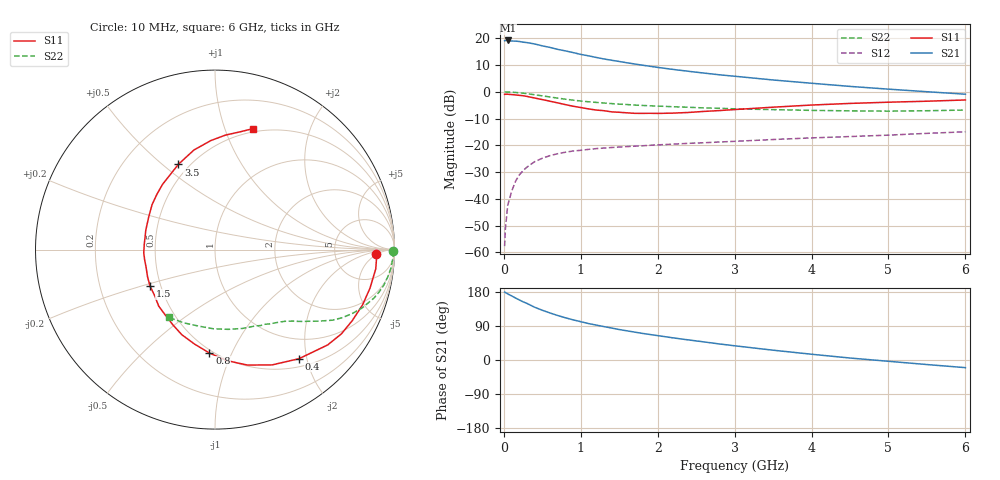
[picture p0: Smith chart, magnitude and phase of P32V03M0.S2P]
! SIEMENS Small Signal Semiconductors
! BFP181
! Si NPN RF Bipolar Junction Transistor in SOT143
! VCE = 2 V  IC = 3 mA
! Common Emitter S-Parameters:  March  1996
# GHz  S  MA  R  50
!  f  S11  S21  S12  S22
! GHz  MAG  ANG  MAG  ANG  MAG  ANG  MAG  ANG
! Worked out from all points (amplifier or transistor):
!   36 points, 10 MHz to 6 GHz, reference 50 ohm
!   highest |S21| = 19.2 dB at 50 MHz (marker M1)
!   |S21| within 3 dB of that: start of sweep to 654.1 MHz
!   unconditionally stable (mu >= 1): 2.041 GHz to end of sweep
!   at 250 MHz: K = 0.16, MSG = 24.0 dB, |S12| = -29.5 dB
!   at 1.4 GHz: K = 0.78, MSG = 16.3 dB, |S12| = -20.8 dB
!   at 6 GHz: K = 1.08, MAG = 5.4 dB, |S12| = -14.9 dB
!   lowest NFmin = 1.40 dB at 450 MHz
!   S11 on the Smith chart (normalised r, x): 10 MHz: 18, -4; 400 MHz: 0.63, -1.86; 800 MHz: 0.48, -0.83; 1.5 GHz: 0.44, -0.21; 3.5 GHz: 0.44, +0.57; 6 GHz: 0.47, +1.25
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0.01  0.8979 -1.5  9.05 179.1  0.0013 89.3  0.9943 -0.6
0.02  0.9013 -3.0  9.13 178.3  0.0027 84.5  0.9957 -1.2
0.05  0.9022 -6.8  9.15 174.5  0.0075 89.4  0.9913 -3.1
0.2  0.861 -27.4  8.767 158.6  0.0279 74.5  0.9609 -11.9
0.25  0.8463 -33.7  8.497 153.5  0.0335 70.7  0.9443 -14.5
0.3  0.8225 -40.2  8.354 149.3  0.0391 67.2  0.9254 -17.0
0.4  0.7672 -52.4  7.867 139.3  0.0494 61.5  0.8833 -21.5
0.5  0.7171 -63.6  7.254 131.3  0.0573 55.7  0.8412 -25.2
0.6  0.6683 -74.3  6.775 124.1  0.0642 51.1  0.8019 -28.3
0.7  0.6222 -83.9  6.236 117.4  0.0697 47.6  0.7635 -31.0
0.8  0.5769 -93.1  5.84 111.4  0.0743 44.5  0.7295 -32.9
0.9  0.5386 -102.2  5.43 106.0  0.0783 41.6  0.7001 -34.7
1.1  0.4802 -119.3  4.72 96.2  0.084 37.8  0.653 -37.7
1.3  0.4444 -134.9  4.127 88.2  0.089 34.7  0.6182 -40.3
1.5  0.4151 -150.7  3.701 80.4  0.0929 32.8  0.5895 -42.5
1.8  0.3961 -171.9  3.157 70.3  0.098 30.9  0.5572 -45.8
2.2  0.4004 164.4  2.629 58.4  0.1052 28.6  0.5269 -50.8
2.8  0.4465 136.6  2.087 42.4  0.1153 26.0  0.4933 -59.1
3.5  0.5168 113.3  1.668 25.9  0.1284 23.6  0.4653 -70.7
4.5  0.6079 92.2  1.265 5.2  0.1459 19.0  0.4413 -91.1
5.5  0.6685 78.4  1.006 -12.0  0.1674 15.2  0.4436 -113.1
6  0.7055 72.7  0.904 -20.2  0.179 12.2  0.4569 -124.3
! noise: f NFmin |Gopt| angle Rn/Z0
0.45  1.4  0.56  17  0.36
0.9  1.5  0.45  35  0.34
1.8  1.85  0.25  82  0.36
